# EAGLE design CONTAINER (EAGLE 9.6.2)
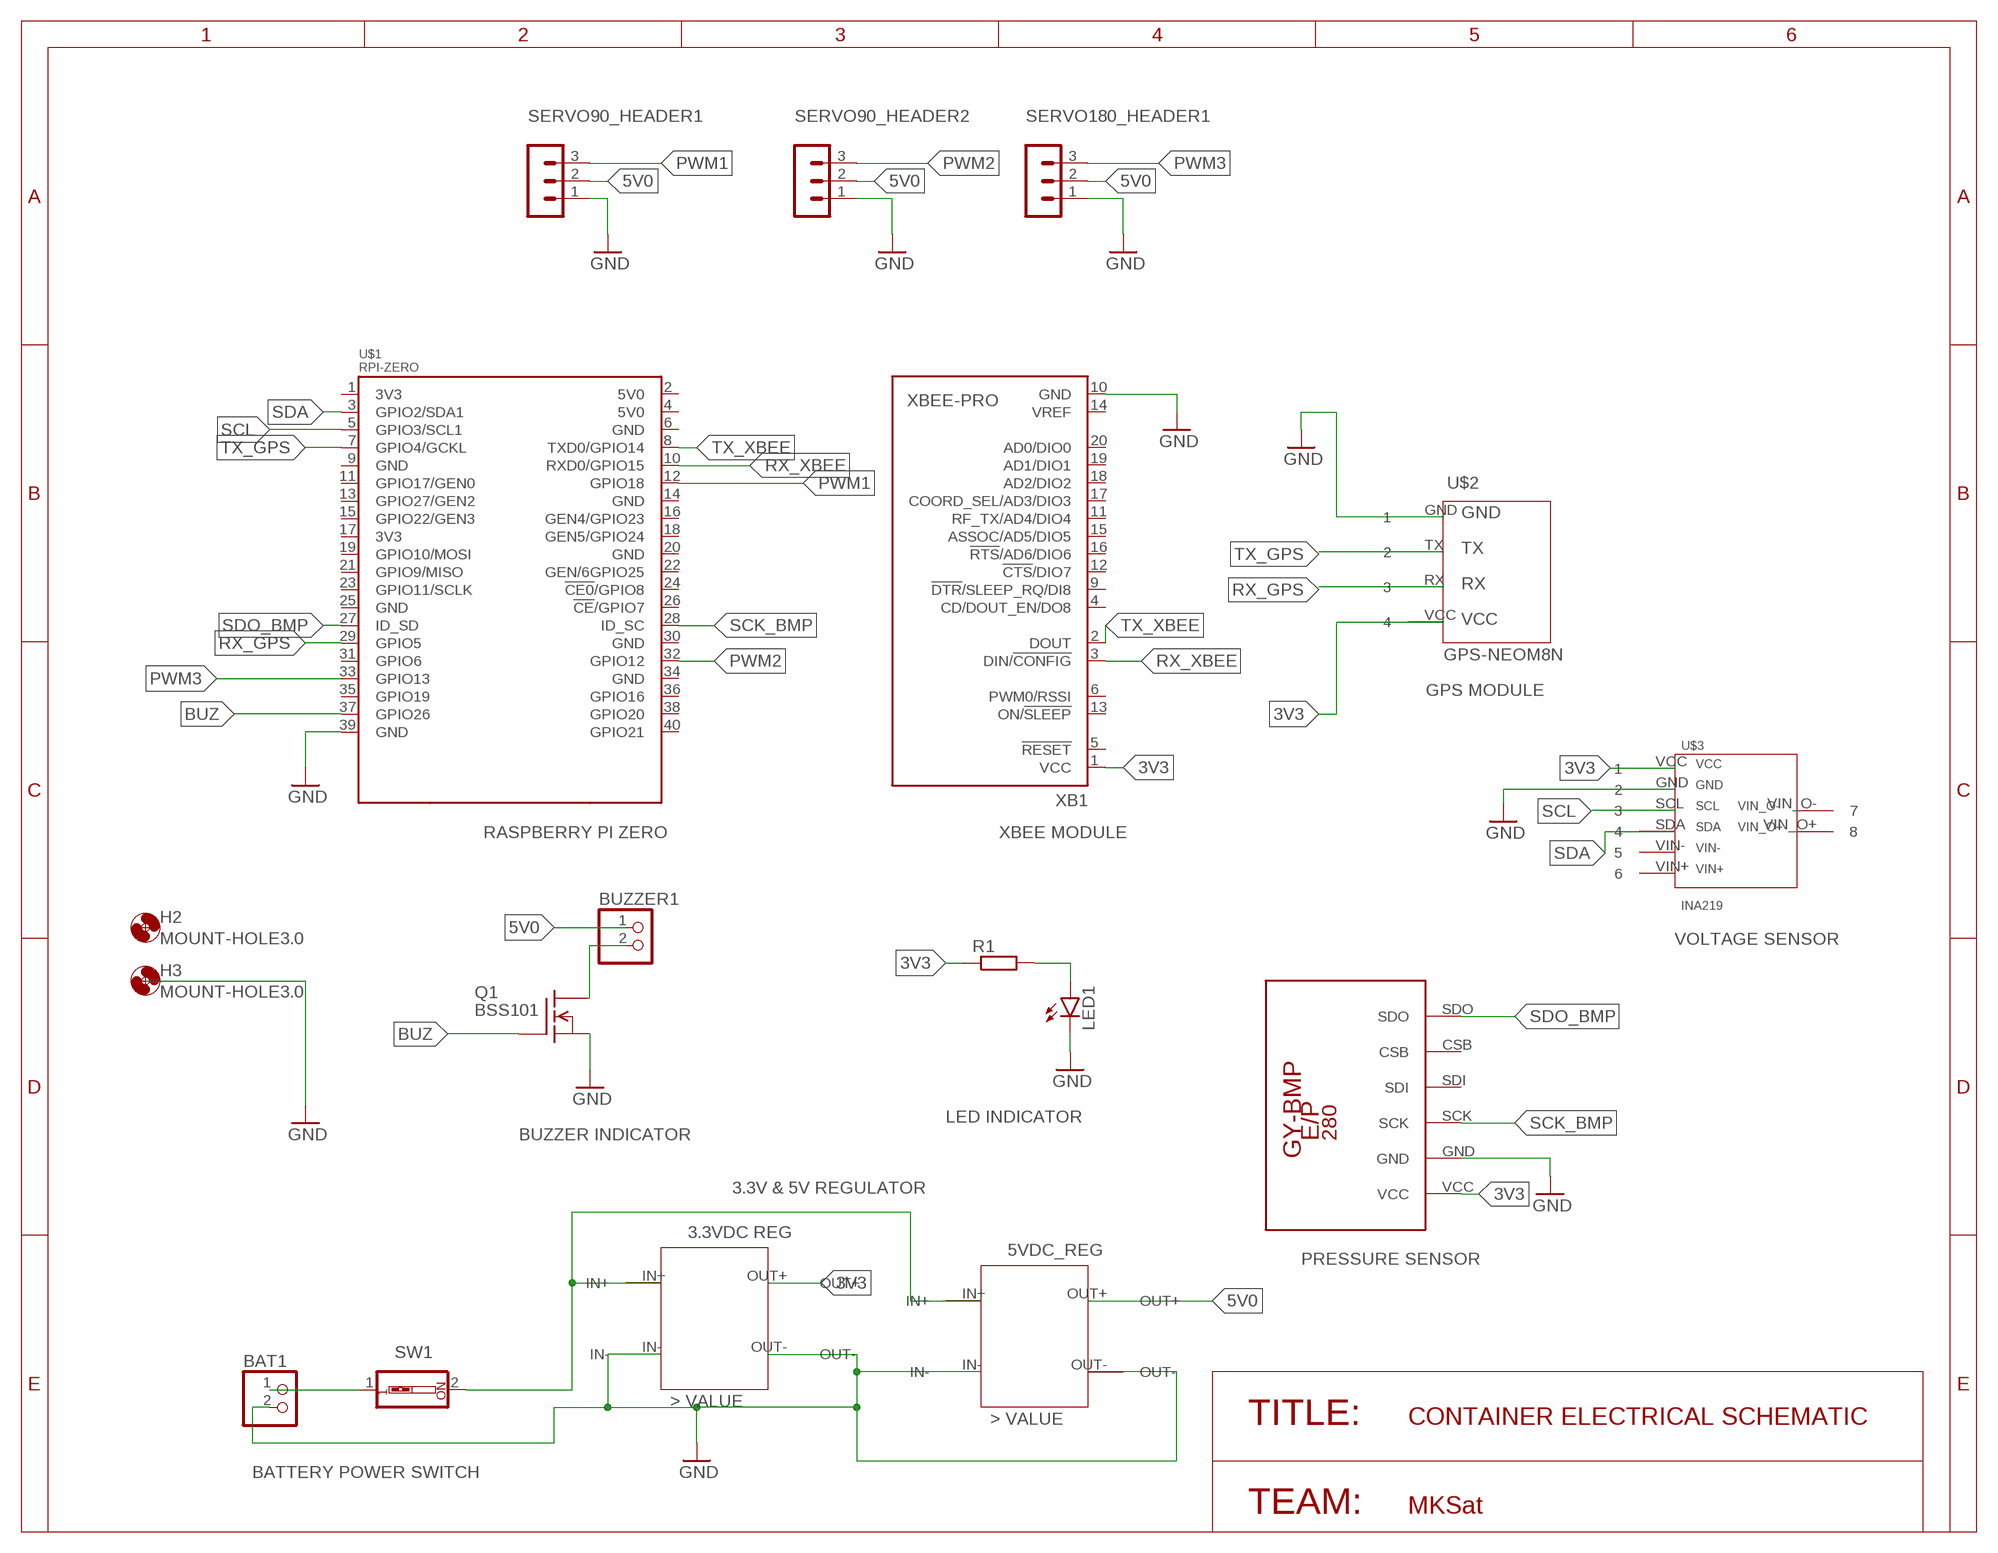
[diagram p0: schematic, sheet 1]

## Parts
BAT1  PINHD-1X2/90  [1X02/90]
BUZZER1  PINHD-1X2/90  [1X02/90]
H2  MOUNT-HOLE3.0  [3,0]
H3  MOUNT-HOLE3.0  [3,0]
LED1  LED5MM  [LED5MM]
Q1  BSS101  [TO92]
R1  R-EU_0207/12  [0207/12]
SERVO90_HEADER1  MA03-1  [MA03-1]
SERVO90_HEADER2  MA03-1  [MA03-1]
SERVO180_HEADER1  MA03-1  [MA03-1]
SW1  SW_DIP-1  [EDG-01]
U$1  RPI-ZERO  [RASPBERRYPI_BASTELSTUBE_V13_RASPI_BOARD_B+_FULL]
U$2  GPS-NEOM8N  [GPS_NEO_M8N]
U$3  INA219  [INA219_LIB]
U$4  GY-BPM280  [GY-BMP280-FOOTPRINT]
U$5  3VDC_REG  [3VDC_REG]
U$6  5VDC_REG  [5VDC_REG]
XB1  XBEE-PRO  [XBEE-PRO]

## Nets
3V3: R1.1 U$2.VCC U$3.VCC U$4.VCC U$5.OUT+ XB1.1(VCC)
5V0: BUZZER1.1 SERVO90_HEADER1.2 SERVO90_HEADER2.2 SERVO180_HEADER1.2 U$6.OUT+
BUZ: Q1.2(G) U$1.37(GPIO26)
GND: BAT1.2 LED1.K(C) Q1.1(S) SERVO90_HEADER1.1 SERVO90_HEADER2.1 SERVO180_HEADER1.1 U$1.39(GND) U$2.GND U$3.GND U$4.GND U$5.IN- U$5.OUT- U$6.IN- U$6.OUT- XB1.10(GND)
N$5: LED1.A R1.2
N$6: BAT1.1 SW1.1
N$7: SW1.2 U$5.IN+ U$6.IN+
N$12: BUZZER1.2 Q1.3(D)
PWM1: SERVO90_HEADER1.3 U$1.12(GPIO18)
PWM2: SERVO90_HEADER2.3 U$1.32(GPIO12)
PWM3: SERVO180_HEADER1.3 U$1.33(GPIO13)
RX_GPS: U$1.29(GPIO5) U$2.RX
RX_XBEE: U$1.10(RXD0/GPIO15) XB1.3(DIN/!CONFIG)
SCK_BMP: U$1.28(ID_SC) U$4.SCK
SCL: U$1.5(GPIO3/SCL1) U$3.SCL
SDA: U$1.3(GPIO2/SDA1) U$3.SDA
SDO_BMP: U$1.27(ID_SD) U$4.SDO
TX_GPS: U$1.7(GPIO4/GCKL) U$2.TX
TX_XBEE: U$1.8(TXD0/GPIO14) XB1.2(DOUT)
Unconnected: U$1.1(3V3) U$1.2(5V0) U$1.4(5V0) U$1.6(GND) U$1.9(GND) U$1.11(GPIO17/GEN0) U$1.13(GPIO27/GEN2) U$1.14(GND) U$1.15(GPIO22/GEN3) U$1.16(GEN4/GPIO23) U$1.17(3V3) U$1.18(GEN5/GPIO24) U$1.19(GPIO10/MOSI) U$1.20(GND) U$1.21(GPIO9/MISO) U$1.22(GEN/6GPIO25) U$1.23(GPIO11/SCLK) U$1.24(!CE0!/GPIO8) U$1.25(GND) U$1.26(!CE!/GPIO7) U$1.30(GND) U$1.31(GPIO6) U$1.34(GND) U$1.35(GPIO19) U$1.36(GPIO16) U$1.38(GPIO20) U$1.40(GPIO21) U$3.VIN+ U$3.VIN- U$3.VIN_O+ U$3.VIN_O- U$4.CSB U$4.SDI XB1.4(CD/DOUT_EN/DO8) XB1.5(!RESET) XB1.6(PWM0/RSSI) XB1.9(!DTR!/SLEEP_RQ/DI8) XB1.11(RF_TX/AD4/DIO4) XB1.12(!CTS!/DIO7) XB1.13(ON/!SLEEP) XB1.14(VREF) XB1.15(ASSOC/AD5/DIO5) XB1.16(!RTS!/AD6/DIO6) XB1.17(COORD_SEL/AD3/DIO3) XB1.18(AD2/DIO2) XB1.19(AD1/DIO1) XB1.20(AD0/DIO0)

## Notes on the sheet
- GPS MODULE
- RASPBERRY PI ZERO | XBEE MODULE
- VOLTAGE SENSOR
- LED INDICATOR
- BUZZER INDICATOR
- 3.3V & 5V REGULATOR
- PRESSURE SENSOR
- TITLE: | CONTAINER ELECTRICAL SCHEMATIC
- BATTERY POWER SWITCH
- TEAM: | MKSat

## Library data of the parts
BAT1 BUZZER1 = pinhead:PINHD-1X2: PIN HEADER
H2 H3 = holes:MOUNT-HOLE: MOUNTING HOLE with drill center marker
LED1 = led:LED: LED
Q1 = transistor-fet:BSS101: N-Channel Enhancement MOSFET 200V; 0,16A; 11Ohm
R1 = rcl:R-EU_: RESISTOR, European symbol; SPICEPREFIX: R
SERVO90_HEADER1 SERVO90_HEADER2 SERVO180_HEADER1 = con-lstb:MA03-1: PIN HEADER; OC_FARNELL: unknown; OC_NEWARK: unknown
SW1 = special:SW_DIP-1: DIP SWITCH
U$1 = RPI-Zero:RPI-ZERO
U$2 = GPS NEO M8N:GPS-NEOM8N
U$3 = INA219_LIB:INA219
U$4 = GY-BMP280:GY-BPM280
U$5 = VOLTAGE_REGULATORS_CANSAT:3VDC_REG
U$6 = VOLTAGE_REGULATORS_CANSAT:5VDC_REG
XB1 = maxstream:XBEE: XBee (TM) /XBee-PRO(TM) OEM RF Modules Source: MaxStream, Inc. xbee_productmanual.pdf; MPN: XBP24-AWI-001; OC_FARNELL: 1337916; OC_NEWARK: 42M2667

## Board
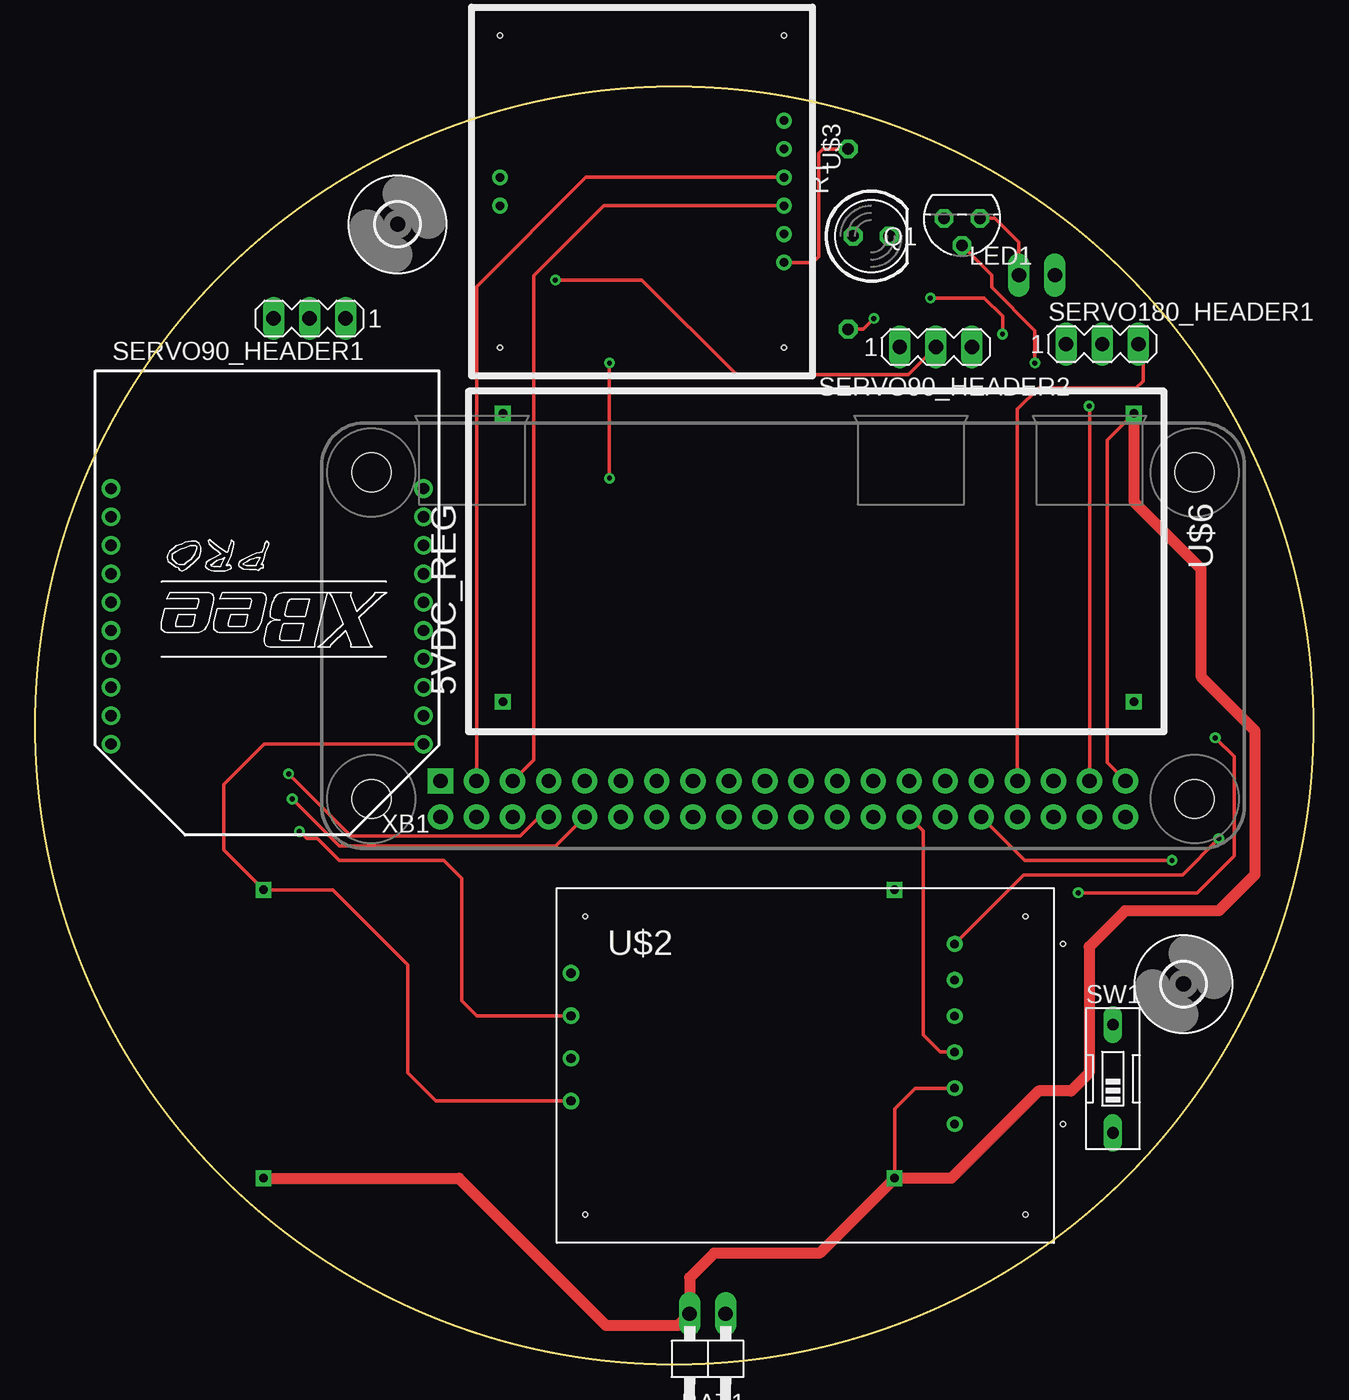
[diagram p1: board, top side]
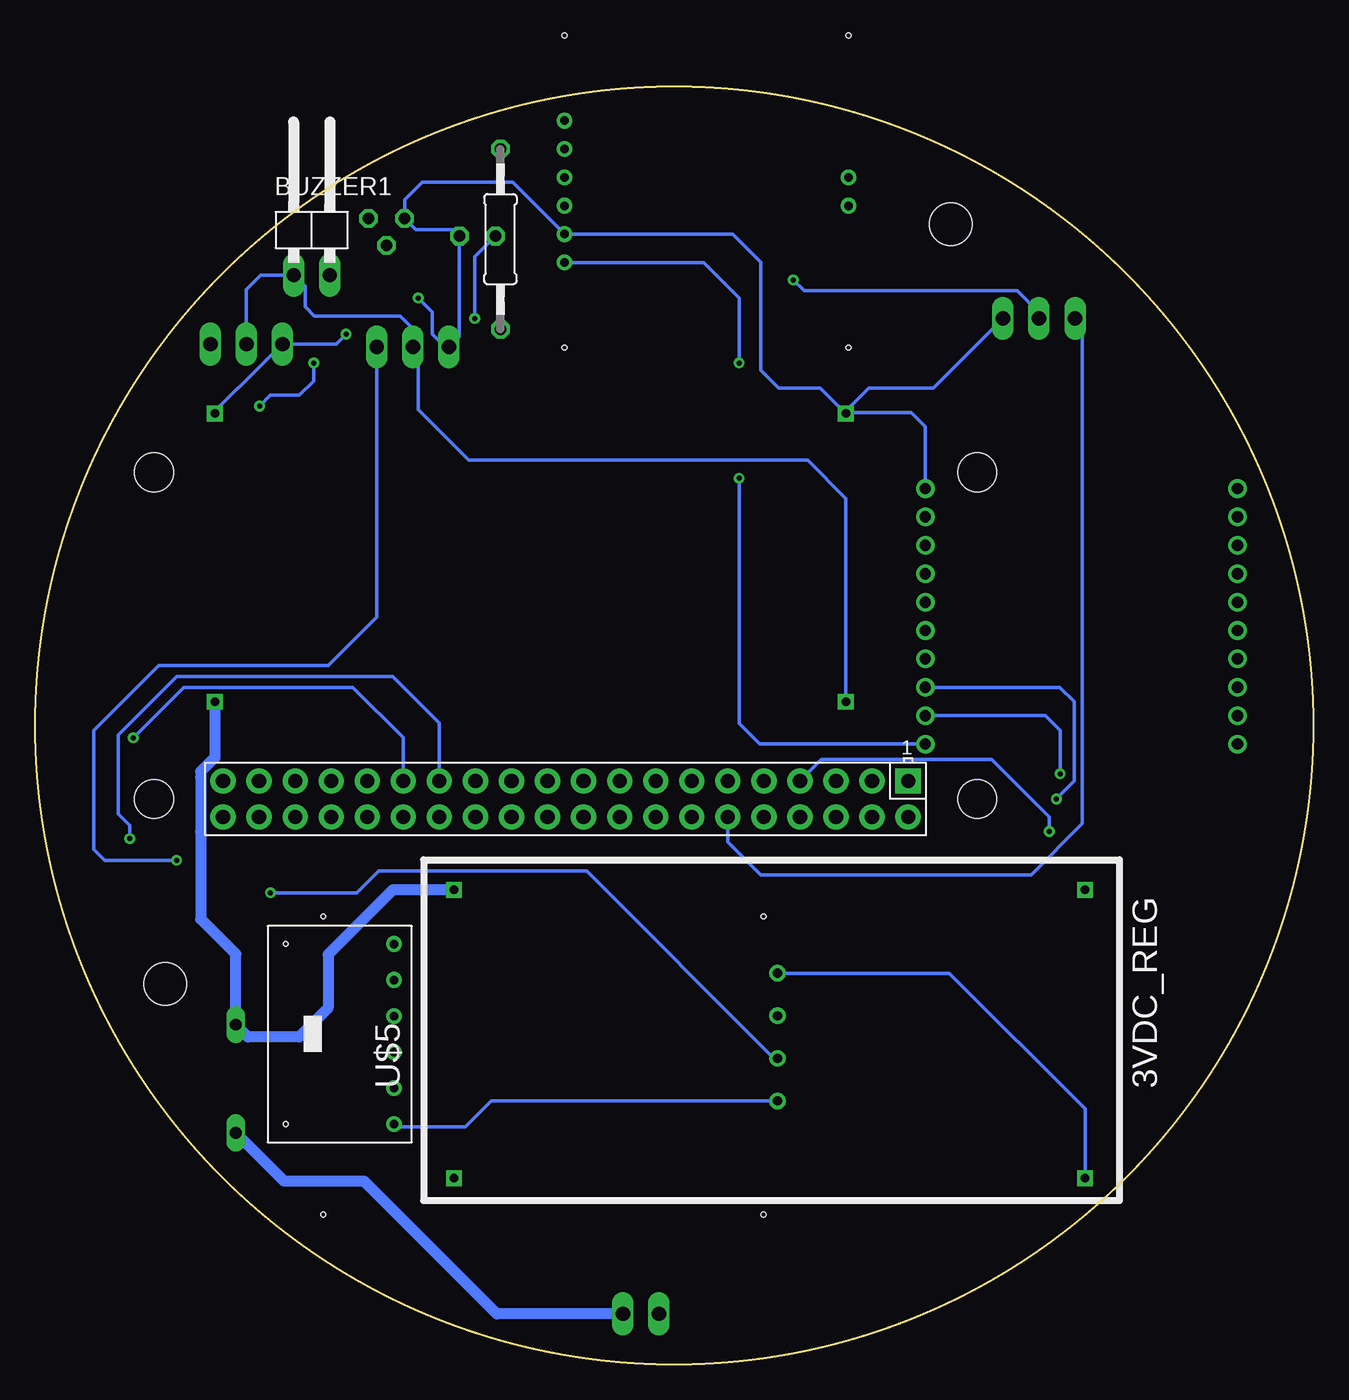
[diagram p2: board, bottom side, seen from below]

Size 90 x 90 mm. Coordinates in mm from the lower left corner, seen from the top.
Outline: circle at 45,45 radius 45
Copper layers (1*16): Top 0.035mm / dielectric 1.5mm / Bottom 0.035mm
Design rules "default *": minimum track width 6mil, minimum drill 0.35mm, track to track 12mil, track to pad 12mil, pad to pad 12mil, via to via 12mil, smd to smd 12mil, copper to edge 40mil, drill to drill 6mil, minimum pad ring 10mil, minimum via ring 8mil, stop-mask expansion 4mil, vias tented up to drill 0mil, thermal gap 10mil

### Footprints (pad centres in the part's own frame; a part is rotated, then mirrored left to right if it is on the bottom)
1X02/90 = drill 1.016 long: 1 -1.27,-3.81; 2 1.27,-3.81
3,0 = hole 3: 0,0
LED5MM = drill 0.813 octagon: A -1.27,0; K 1.27,0
TO92 = drill 0.813 octagon: 1 1.27,0; 2 0,1.905; 3 -1.27,0
0207/12 = drill 0.813 octagon: 1 -6.35,0; 2 6.35,0
MA03-1 = drill 1.016 long: 1 -2.54,0; 2 0,0; 3 2.54,0
EDG-01 = drill 0.813 long: 1 0,-3.81; 2 0,3.81
RASPBERRYPI_BASTELSTUBE_V13_RASPI_BOARD_B+_FULL = drill 1 pad 1.778 square: 1 8.37,25.23 | drill 1 pad 1.778: 2 8.37,27.77; 3 10.91,25.23; 4 10.91,27.77; 5 13.45,25.23; 6 13.45,27.77; 7 15.99,25.23; 8 15.99,27.77; 9 18.53,25.23; 10 18.53,27.77; 11 21.07,25.23; 12 21.07,27.77; 13 23.61,25.23; 14 23.61,27.77; 15 26.15,25.23; 16 26.15,27.77; 17 28.69,25.23; 18 28.69,27.77; 19 31.23,25.23; 20 31.23,27.77; 21 33.77,25.23; 22 33.77,27.77; 23 36.31,25.23; 24 36.31,27.77; 25 38.85,25.23; 26 38.85,27.77; 27 41.39,25.23; 28 41.39,27.77; 29 43.93,25.23; 30 43.93,27.77; 31 46.47,25.23; 32 46.47,27.77; 33 49.01,25.23; 34 49.01,27.77; 35 51.55,25.23; 36 51.55,27.77; 37 54.09,25.23; 38 54.09,27.77; 39 56.63,25.23; 40 56.63,27.77 | hole 2.75: 3.5,3.5; 3.5,26.5; 61.5,3.5; 61.5,26.5
GPS_NEO_M8N = drill 0.65: GND -15.27,6.54; RX -15.27,0.54; TX -15.27,3.54; VCC -15.27,-2.46 | hole 0.35: -14.27,10.54; 16.73,10.54; -14.27,-10.46; 16.73,-10.46
INA219_LIB = drill 0.6: GND -10,4; SCL -10,2; SDA -10,0; VCC -10,6; VIN+ -10,-4; VIN- -10,-2; VIN_O+ 10,0; VIN_O- 10,2 | hole 0.35: -10,12; 10,12; -10,-10; 10,-10
GY-BMP280-FOOTPRINT = drill 0.6: CSB 11.43,0; GND 3.81,0; SCK 6.35,0; SDI 8.89,0; SDO 13.97,0; VCC 1.27,0 | hole 0.35: 1.27,7.62; 13.97,7.62
3VDC_REG = drill 0.6 square: IN+ -22.86,8.89; IN- -22.86,-11.43; OUT+ 21.59,8.89; OUT- 21.59,-11.43
5VDC_REG = drill 0.6 square: IN+ -22.86,8.89; IN- -22.86,-11.43; OUT+ 21.59,8.89; OUT- 21.59,-11.43
XBEE-PRO = drill 0.8 pad 1.27: 1 -11,9; 2 -11,7; 3 -11,5; 4 -11,3; 5 -11,1; 6 -11,-1; 7 -11,-3; 8 -11,-5; 9 -11,-7; 10 -11,-9; 11 11,-9; 12 11,-7; 13 11,-5; 14 11,-3; 15 11,-1; 16 11,1; 17 11,3; 18 11,5; 19 11,7; 20 11,9

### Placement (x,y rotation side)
BAT1  47.35,-0.27 180 top
BUZZER1  70.54,80.54 0 bottom
H2  25.51,80.32 0 top
H3  80.87,26.78 0 top
LED1  58.87,79.48 0 top
Q1  65.27,80.73 180 top
R1  57.25,79.27 270 bottom
SERVO90_HEADER1  19.31,73.68 180 top
SERVO90_HEADER2  63.42,71.67 0 top
SERVO180_HEADER1  75.15,71.87 0 top
SW1  75.89,20.1 0 top
U$1  20.16,66.32 180 bottom
U$2  53,21 0 top
U$3  42.73,83.62 180 top
U$4  64.75,15.63 90 bottom
U$5  37.65,24.52 0 bottom
U$6  54.51,55.55 180 top
XB1  16.32,52.69 180 top

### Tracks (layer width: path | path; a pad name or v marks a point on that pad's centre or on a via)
3V3  (via drill 0.35)
  Top 0.254: U$3.VCC 54.76,77.62 55.17,78.02 55.17,85.31 55.47,85.62 55.98,85.62 R1.1 | U$2.VCC 28.18,18.54 26.21,20.51 26.21,28.13 20.93,33.41 U$5.OUT+ 13.26,36.22 13.26,40.83 16.12,43.69 XB1.1 | v40.43,62.42 v40.43,70.55
  Bottom 0.254: U$2.VCC 57.9,18.54 59.74,16.7 64.55,16.7 U$4.VCC | XB1.1 38.98,43.69 40.43,45.15 v40.43,62.42 | v40.43,70.55 40.43,75.12 42.93,77.62 U$3.VCC
5V0  (via drill 0.35)
  Top 0.254: v36.62,76.39 42.72,76.39 49.4,69.71 61.46,69.71 SERVO90_HEADER2.2
  Bottom 0.254: SERVO180_HEADER1.2 75.15,75.71 74.13,76.73 BUZZER1.1 71.76,76.73 71,75.97 71,74.5 70.35,73.85 64.31,73.85 63.42,72.96 SERVO90_HEADER2.2 63.04,71.29 63.04,67.25 59.48,63.69 35.61,63.69 32.92,61 U$6.OUT+ | SERVO90_HEADER1.2 19.31,74.1 20.85,75.63 23.11,75.63 35.86,75.63 v36.62,76.39
BUZ  (via drill 0.35)
  Top 0.254: U$1.37 74.25,67.47 v74.22,67.5 | Q1.2 67.36,76.74 67.36,75.88 70.41,72.83 v70.41,70.55
  Bottom 0.254: v70.41,70.55 70.41,69.28 71.42,68.26 73.45,68.26 v74.22,67.5
GND  (via drill 0.35)
  Top 0.254: v68.12,72.58 68.12,73.85 66.85,75.12 v63.04,75.12 | U$5.IN- 60.51,17.98 61.97,19.44 U$4.GND | U$1.39 75.49,42.39 75.49,65.1 U$6.IN-
  Top 0.762: U$6.IN- 77.37,60.79 82.09,56.07 82.09,48.45 85.9,44.64 85.9,34.48 83.36,31.94 76.76,31.94 74.22,29.4 74.22,20.51 72.95,19.24 70.66,19.24 64.51,13.09 U$5.IN- 55.23,7.81 47.8,7.81 46.08,6.09 BAT1.2 45.27,2.73 40.18,2.73 29.82,13.09 U$5.OUT-
  Bottom 0.254: v68.12,72.58 68.83,71.87 SERVO180_HEADER1.1 75.71,68.77 75.74,68.77 77.37,67.14 U$6.IN- | v63.04,75.12 62.03,74.11 62.03,72.57 61.13,71.67 SERVO90_HEADER2.1 60.14,72.41 LED1.K 60.61,79.95 63.22,79.95 Q1.1 64,82.03 62.76,83.27 56.38,83.27 U$3.GND 40.87,79.62 38.91,77.66 38.91,70.04 37.64,68.77 34.71,68.77 33,67.06 | U$2.GND 25.62,27.54 16.06,17.98 U$5.OUT- | 33,67.06 U$6.OUT- 32.92,67.14 31.29,68.77 26.76,68.77 SERVO90_HEADER1.1 | XB1.10 27.32,66.07 28.31,67.06 33,67.06
N$5  (via drill 0.35)
  Top 0.254: R1.2 58.3,72.92 v59.06,73.68
  Bottom 0.254: v59.06,73.68 59.06,78.02 LED1.A
N$6
  Bottom 0.762: BAT1.1 57.5,3.54 66.85,12.89 72.49,12.89 SW1.1
N$7
  Bottom 0.762: U$6.IN+ 77.37,42.74 78.36,41.74 78.36,41.34 78.36,37.53 78.36,31.36 75.89,28.89 SW1.2 75.03,23.05 71.42,23.05 69.39,25.08 69.39,28.85 64.83,33.41 U$5.IN+
N$12
  Top 0.254: BUZZER1.2 69.27,79.05 67.59,80.73 Q1.3
PWM1
  Bottom 0.254: SERVO90_HEADER1.3 16.26,73.17 16.26,38.08 19.86,34.48 38.91,34.48 41.23,36.8 U$1.12
PWM2  (via drill 0.35)
  Top 0.254: U$1.32 69.68,35.5 v80.06,35.5
  Bottom 0.254: SERVO90_HEADER2.3 65.96,52.64 69.39,49.21 81.33,49.21 85.9,44.64 85.9,36.26 85.14,35.5 v80.06,35.5
PWM3
  Top 0.254: U$1.33 69.17,67.28 70.66,68.77 77.52,68.77 78.03,69.28 78.03,71.53 SERVO180_HEADER1.3
RX_GPS  (via drill 0.35)
  Top 0.254: v73.45,33.21 81.84,33.21 84.43,35.81 84.43,42.81 v83.11,44.13
  Bottom 0.254: U$2.RX 37.98,21.54 51.18,34.73 65.83,34.73 67.36,33.21 v73.45,33.21 | U$1.29 64.09,44.14 67.64,47.69 79.55,47.69 v83.11,44.13
RX_XBEE  (via drill 0.35)
  Top 0.254: U$1.10 36.65,36.51 21.38,36.51 v18.08,39.81
  Bottom 0.254: v18.08,39.81 16.82,41.08 16.82,46.67 17.84,47.69 XB1.3
SCK_BMP
  Top 0.254: U$1.28 62.53,37.57 62.53,23.19 63.74,21.98 U$4.SCK
SCL
  Top 0.254: U$3.SCL 40.03,81.62 35.1,76.69 35.1,45.15 35.1,42.58 U$1.5
SDA
  Top 0.254: U$3.SDA 38.76,83.62 31.07,75.93 U$1.3
SDO_BMP  (via drill 0.35)
  Top 0.254: v83.36,37.02 80.82,34.48 69.63,34.48 U$4.SDO
  Bottom 0.254: U$1.27 61.55,45.18 64.82,48.45 80.06,48.45 84.18,44.33 84.18,38.78 83.36,37.96 v83.36,37.02
TX_GPS  (via drill 0.35)
  Top 0.254: v18.59,37.53 19.1,37.02 19.86,37.02 21.38,35.5 28.75,35.5 30.02,34.23 30.02,25.59 31.07,24.54 U$2.TX
  Bottom 0.254: U$1.7 34.64,42.6 22.65,42.6 18.59,38.54 v18.59,37.53
TX_XBEE  (via drill 0.35)
  Top 0.254: U$1.8 35.48,38.55 34.16,37.23 22.19,37.23 v17.83,41.59
  Bottom 0.254: v17.83,41.59 17.83,44.64 18.88,45.69 XB1.2

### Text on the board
Text: BMP-280 | INA-219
